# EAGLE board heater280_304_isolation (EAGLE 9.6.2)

No outline drawn. Coordinates in mm, seen from the top.
Copper layers (1*16): Top 0.035mm / dielectric 1.5mm / Bottom 0.035mm
Design rules "default": minimum track width 6mil, minimum drill 0.35mm, track to track 6mil, track to pad 6mil, pad to pad 6mil, via to via 6mil, smd to smd 6mil, copper to edge 40mil, drill to drill 6mil, minimum pad ring 10mil, minimum via ring 8mil, stop-mask expansion 4mil, vias tented up to drill 0mil, thermal gap 10mil

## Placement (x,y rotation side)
U$1  [CE-4MM]  0.84,194.13 0 top

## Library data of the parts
U$1 = logo

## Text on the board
tPlace: ECS, Am Wenigerflur 14, 54498 Piesport | HEATER280_304 | ISOLATION PLATE / (END PLATE)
